(* Logix 5000 AddOnInstructionDefinition export YAI_Assy_151_116_EIP_Hz; software revision 21.03 *)

ADD_ON_INSTRUCTION YAI_Assy_151_116_EIP_Hz   (* revision 1.1, vendor Yaskawa America, Inc. *)
// YAI Assembly 151 and 116
// Help:
// This add-on instruction is for use with input assemblie 166 and output assemblies 116.
// Node_Input_Assy is defined as the node's input assembly integer array.
// Node_Output_Assy is defined as the node's output assembly integer array.
// Torque limit/reference, torque compensation and torque output variables are only available with A1000.
VAR_IN_OUT
   Node_Input_Assy : AB:ETHERNET_MODULE_INT_8Bytes:I:0; {required}   // Input assembly words
   Node_Output_Assy : AB:ETHERNET_MODULE_INT_44Bytes:O:0; {required}   // Output assembly words
END_VAR
VAR_INPUT
   RunFwd : BOOL; {visible}   // Forward run command
   RunRev : BOOL; {visible}   // Reverse run command
   MFI_3 : BOOL; {visible}   // Multi-function input 3
   MFI_4 : BOOL; {visible}   // Multi-function input 4
   MFI_5 : BOOL; {visible}   // Multi-function input 5
   MFI_6 : BOOL; {visible}   // Multi-function input 6
   MFI_7 : BOOL; {visible}   // Multi-function input 7
   MFI_8 : BOOL; {visible}   // Multi-function input 8
   External_Fault : BOOL;   // External fault command (EF0)
   FaultReset : BOOL; {visible}   // Fault reset command
   MFO_1 : BOOL; {visible}   // Multi-function output (M1-M2 for A/P1000, MA/MB/MC for V1000)
   MFO_2 : BOOL; {visible}   // Multi-function output (M3-M4 for A/P1000, P1 for V1000)
   MFO_3 : BOOL; {visible}   // Multi-function output (M5-M6 for A/P1000, P2 for V1000)
   Freq_Ref : REAL; {visible}   // Frequency reference command in Hz (xx.xx resolution)
   Torq_Ref_Limit : REAL; {visible}   // Torque reference/limit (A1000 only)
   Torq_Comp : REAL; {visible}   // Torque compensation command (A1000 only)
   Analog_Output_1 : REAL;   // Analog output 1 level command
   Analog_Output_2 : REAL;   // Analog output 2 level command
   Digital_Output_1 : BOOL;   // Digital output 1 activation - M1-M2
   Digital_Output_2 : BOOL;   // Digital output 2 activation - M3-M4
   Digital_Output_3 : BOOL;   // Digital output 3 activation - M5-M6
   Digital_Output_Fault_Enable : BOOL;   // Bit to enable control of fault output relay over the network
   Digital_Output_Fault : BOOL;   // Fault relay activation - MA-MB-MC
   Custom_Out_1 : INT; {visible}   // Custom output 1 - F7-23
   Custom_Out_2 : INT; {visible}   // Custom output 2 - F7-24
   Custom_Out_3 : INT; {visible}   // Custom output 3 - F7-25
   Custom_Out_4 : INT;   // Custom output 4 - F7-26
   Custom_Out_5 : INT;   // Custom output 5 - F7-27
   Custom_Out_6 : INT;   // Custom output 6 - F7-28
   Custom_Out_7 : INT;   // Custom output 7 - F7-29
   Custom_Out_8 : INT;   // Custom output 8 - F7-30
   Custom_Out_9 : INT;   // Custom output 9 - F7-31
   Custom_Out_10 : INT;   // Custom output 10 - F7-32
END_VAR
VAR_OUTPUT
   RunningRev : BOOL; {access Read Only, visible}   // Drive running reverse status bit
   At_Speed : BOOL; {access Read Only, visible}   // Drive at commanded speed status bit
   Ready : BOOL; {access Read Only, visible}   // Drive ready status bit
   Alarm : BOOL; {access Read Only, visible}   // Drive alarm status bit
   Faulted : BOOL; {access Read Only, visible}   // Drive faulted status bit
   Output_Freq : REAL; {access Read Only, visible}   // Drive output frequency in Hz (xx.xx resolution)
   Warning : BOOL; {access Read Only}
   RunningFwd : BOOL; {access Read Only}
END_VAR
VAR_INPUT
   Motor_Rated_Torq : REAL;
END_VAR
VAR_OUTPUT
   Running : BOOL; {access Read Only}
   ZSP : BOOL; {access Read Only}
   Reset : BOOL; {access Read Only}
   OPE : BOOL; {access Read Only}
   UV : BOOL; {access Read Only}
   MFO_1_Status : BOOL; {access Read Only}
   MFO_2_Status : BOOL; {access Read Only}
   MFO_3_Status : BOOL; {access Read Only}
   ZSV : BOOL; {access Read Only}
   Torque_Actual : REAL; {access Read Only}
   Output_Current : REAL; {access Read Only}
END_VAR
VAR_INPUT
   Net_Ref : BOOL;
   Net_Control : BOOL;
END_VAR
VAR_OUTPUT
   NetCtrlStatus : BOOL; {access Read Only}
END_VAR
VAR
   FRef_Convert : DINT;
   FOut_Convert : REAL;
   FOut_Temp : REAL;
   TRef_Convert : INT;
   TComp_Convert : INT;
   IOut_Temp : REAL;
   IOut_Convert : REAL;
   AO1_Convert : INT;
   AO2_Convert : INT;
   Motor_Speed_Temp : REAL;
   Motor_Speed_Convert : REAL;
   Freq_Cmd_Temp : REAL;
   Freq_Cmd_Convert : REAL;
   AI1_Temp : REAL;
   AI1_Convert : REAL;
   DriveStatusTempBits : INT;
   TOut_Temp : REAL;
   TOut_Convert : REAL;
END_VAR

ROUTINE Logic   (* ladder *)
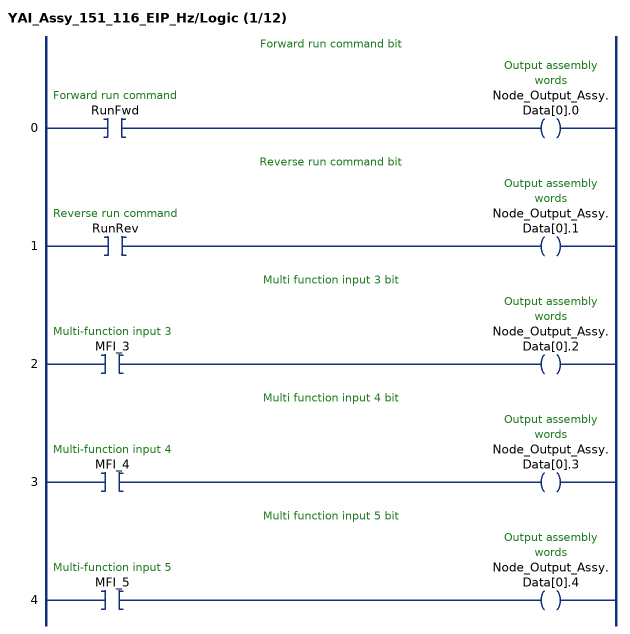
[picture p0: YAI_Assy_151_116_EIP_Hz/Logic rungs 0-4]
   // Forward run command bit
   0: XIC(RunFwd)OTE(Node_Output_Assy.Data[0].0);
   // Reverse run command bit
   1: XIC(RunRev)OTE(Node_Output_Assy.Data[0].1);
   // Multi function input 3 bit
   2: XIC(MFI_3)OTE(Node_Output_Assy.Data[0].2);
   // Multi function input 4 bit
   3: XIC(MFI_4)OTE(Node_Output_Assy.Data[0].3);
   // Multi function input 5 bit
   4: XIC(MFI_5)OTE(Node_Output_Assy.Data[0].4);
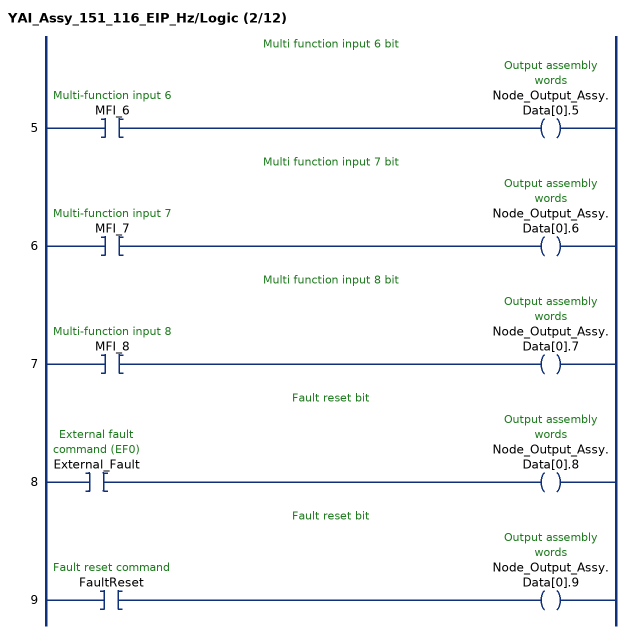
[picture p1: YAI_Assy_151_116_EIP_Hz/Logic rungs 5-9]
   // Multi function input 6 bit
   5: XIC(MFI_6)OTE(Node_Output_Assy.Data[0].5);
   // Multi function input 7 bit
   6: XIC(MFI_7)OTE(Node_Output_Assy.Data[0].6);
   // Multi function input 8 bit
   7: XIC(MFI_8)OTE(Node_Output_Assy.Data[0].7);
   // Fault reset bit
   8: XIC(External_Fault)OTE(Node_Output_Assy.Data[0].8);
   // Fault reset bit
   9: XIC(FaultReset)OTE(Node_Output_Assy.Data[0].9);
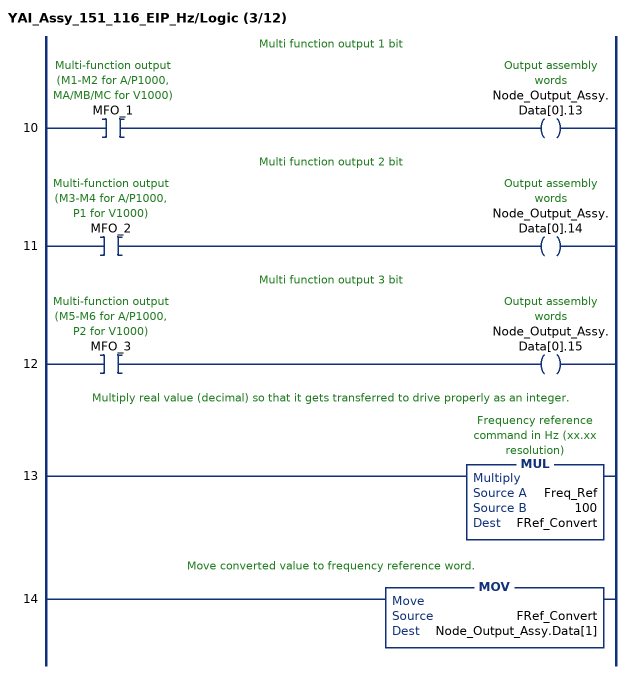
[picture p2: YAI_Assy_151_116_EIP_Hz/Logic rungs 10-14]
   // Multi function output 1 bit
   10: XIC(MFO_1)OTE(Node_Output_Assy.Data[0].13);
   // Multi function output 2 bit
   11: XIC(MFO_2)OTE(Node_Output_Assy.Data[0].14);
   // Multi function output 3 bit
   12: XIC(MFO_3)OTE(Node_Output_Assy.Data[0].15);
   // Multiply real value (decimal) so that it gets transferred to drive properly as an integer.
   13: MUL(Freq_Ref,100,FRef_Convert);
   // Move converted value to frequency reference word.
   14: MOV(FRef_Convert,Node_Output_Assy.Data[1]);
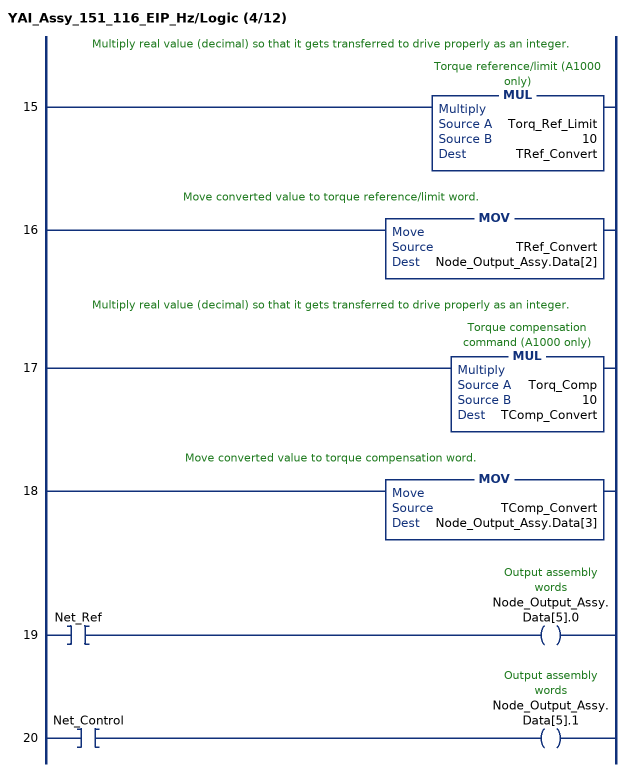
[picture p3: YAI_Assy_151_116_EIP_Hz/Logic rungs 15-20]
   // Multiply real value (decimal) so that it gets transferred to drive properly as an integer.
   15: MUL(Torq_Ref_Limit,10,TRef_Convert);
   // Move converted value to torque reference/limit word.
   16: MOV(TRef_Convert,Node_Output_Assy.Data[2]);
   // Multiply real value (decimal) so that it gets transferred to drive properly as an integer.
   17: MUL(Torq_Comp,10,TComp_Convert);
   // Move converted value to torque compensation word.
   18: MOV(TComp_Convert,Node_Output_Assy.Data[3]);
   19: XIC(Net_Ref)OTE(Node_Output_Assy.Data[5].0);
   20: XIC(Net_Control)OTE(Node_Output_Assy.Data[5].1);
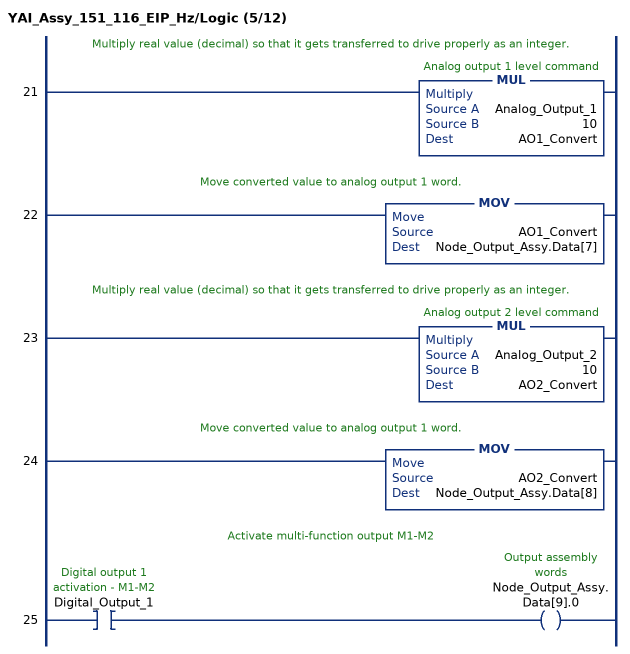
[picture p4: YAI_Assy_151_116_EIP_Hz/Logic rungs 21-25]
   // Multiply real value (decimal) so that it gets transferred to drive properly as an integer.
   21: MUL(Analog_Output_1,10,AO1_Convert);
   // Move converted value to analog output 1 word.
   22: MOV(AO1_Convert,Node_Output_Assy.Data[7]);
   // Multiply real value (decimal) so that it gets transferred to drive properly as an integer.
   23: MUL(Analog_Output_2,10,AO2_Convert);
   // Move converted value to analog output 1 word.
   24: MOV(AO2_Convert,Node_Output_Assy.Data[8]);
   // Activate multi-function output M1-M2
   25: XIC(Digital_Output_1)OTE(Node_Output_Assy.Data[9].0);
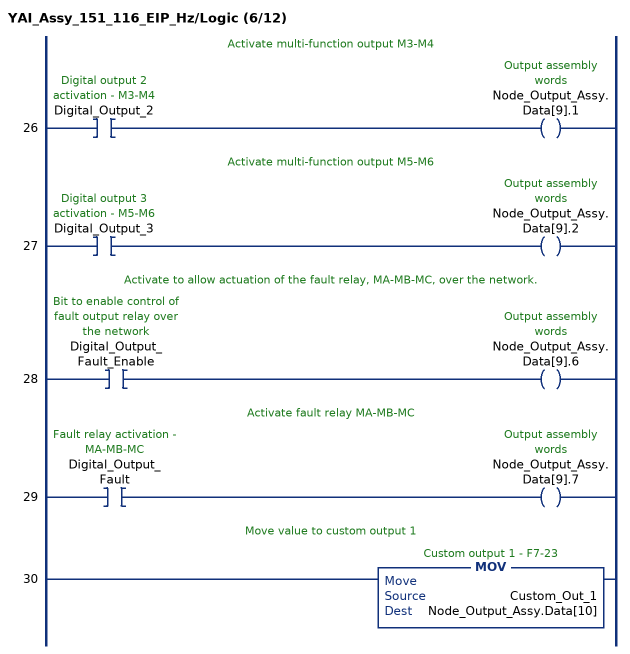
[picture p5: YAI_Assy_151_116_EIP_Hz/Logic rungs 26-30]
   // Activate multi-function output M3-M4
   26: XIC(Digital_Output_2)OTE(Node_Output_Assy.Data[9].1);
   // Activate multi-function output M5-M6
   27: XIC(Digital_Output_3)OTE(Node_Output_Assy.Data[9].2);
   // Activate to allow actuation of the fault relay, MA-MB-MC, over the network.
   28: XIC(Digital_Output_Fault_Enable)OTE(Node_Output_Assy.Data[9].6);
   // Activate fault relay MA-MB-MC
   29: XIC(Digital_Output_Fault)OTE(Node_Output_Assy.Data[9].7);
   // Move value to custom output 1
   30: MOV(Custom_Out_1,Node_Output_Assy.Data[10]);
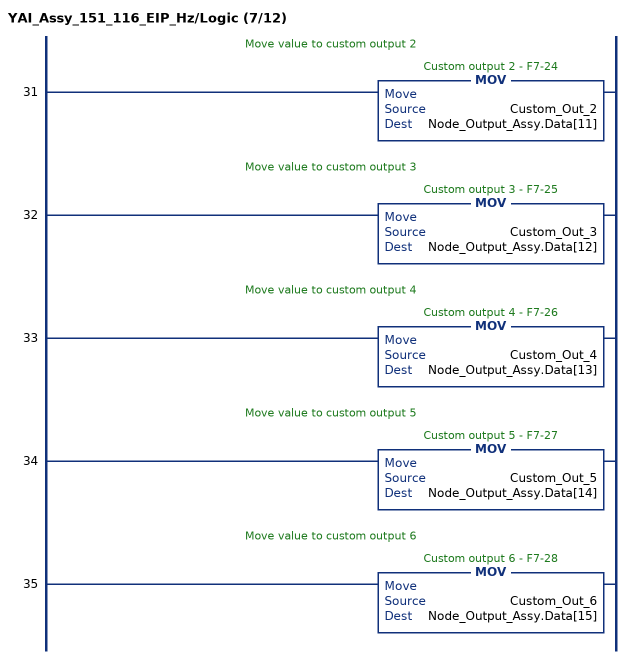
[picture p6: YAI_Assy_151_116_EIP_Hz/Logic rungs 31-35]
   // Move value to custom output 2
   31: MOV(Custom_Out_2,Node_Output_Assy.Data[11]);
   // Move value to custom output 3
   32: MOV(Custom_Out_3,Node_Output_Assy.Data[12]);
   // Move value to custom output 4
   33: MOV(Custom_Out_4,Node_Output_Assy.Data[13]);
   // Move value to custom output 5
   34: MOV(Custom_Out_5,Node_Output_Assy.Data[14]);
   // Move value to custom output 6
   35: MOV(Custom_Out_6,Node_Output_Assy.Data[15]);
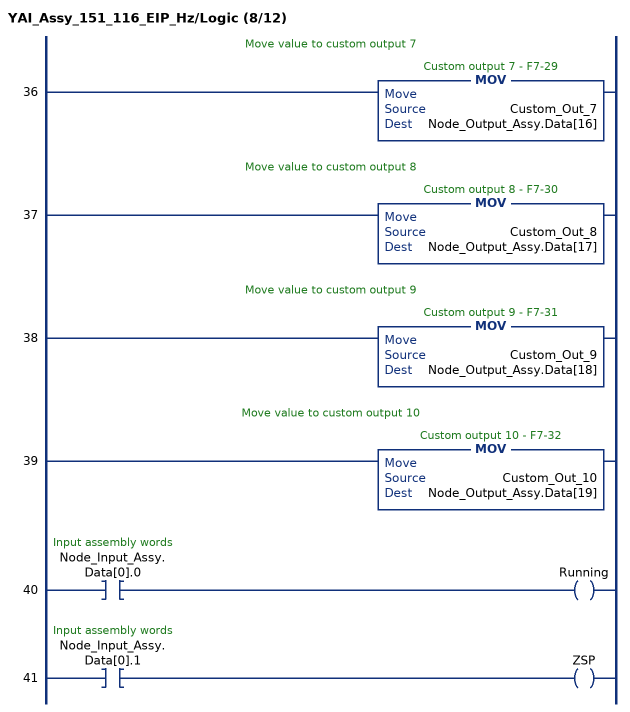
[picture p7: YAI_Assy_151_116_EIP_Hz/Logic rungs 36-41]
   // Move value to custom output 7
   36: MOV(Custom_Out_7,Node_Output_Assy.Data[16]);
   // Move value to custom output 8
   37: MOV(Custom_Out_8,Node_Output_Assy.Data[17]);
   // Move value to custom output 9
   38: MOV(Custom_Out_9,Node_Output_Assy.Data[18]);
   // Move value to custom output 10
   39: MOV(Custom_Out_10,Node_Output_Assy.Data[19]);
   40: XIC(Node_Input_Assy.Data[0].0)OTE(Running);
   41: XIC(Node_Input_Assy.Data[0].1)OTE(ZSP);
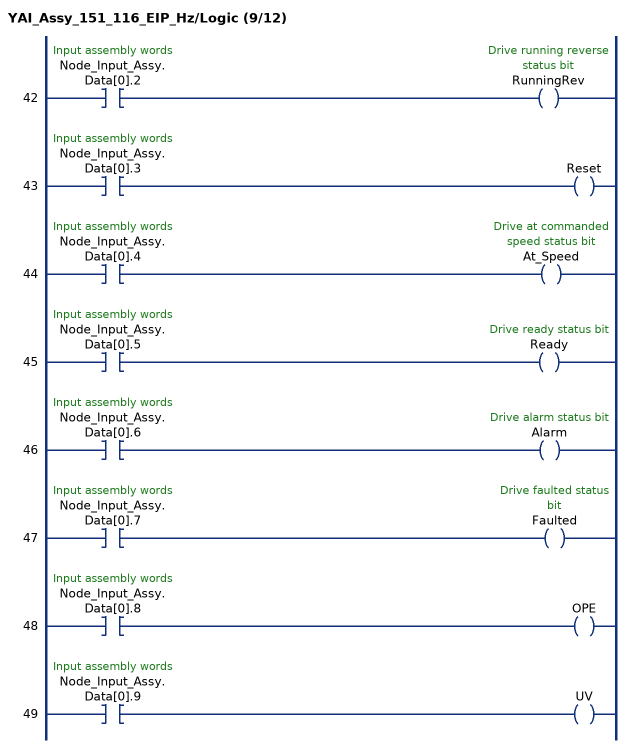
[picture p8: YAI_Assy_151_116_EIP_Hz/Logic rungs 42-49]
   42: XIC(Node_Input_Assy.Data[0].2)OTE(RunningRev);
   43: XIC(Node_Input_Assy.Data[0].3)OTE(Reset);
   44: XIC(Node_Input_Assy.Data[0].4)OTE(At_Speed);
   45: XIC(Node_Input_Assy.Data[0].5)OTE(Ready);
   46: XIC(Node_Input_Assy.Data[0].6)OTE(Alarm);
   47: XIC(Node_Input_Assy.Data[0].7)OTE(Faulted);
   48: XIC(Node_Input_Assy.Data[0].8)OTE(OPE);
   49: XIC(Node_Input_Assy.Data[0].9)OTE(UV);
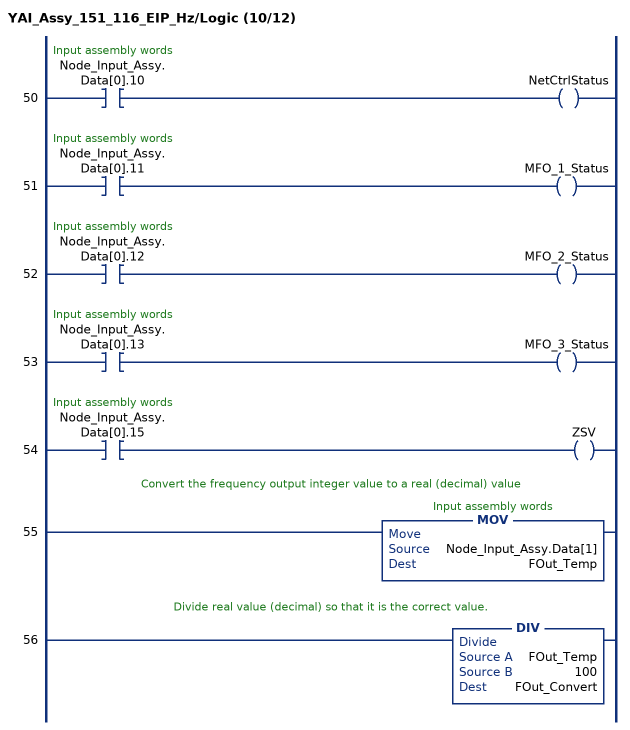
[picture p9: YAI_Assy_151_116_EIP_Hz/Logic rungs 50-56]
   50: XIC(Node_Input_Assy.Data[0].10)OTE(NetCtrlStatus);
   51: XIC(Node_Input_Assy.Data[0].11)OTE(MFO_1_Status);
   52: XIC(Node_Input_Assy.Data[0].12)OTE(MFO_2_Status);
   53: XIC(Node_Input_Assy.Data[0].13)OTE(MFO_3_Status);
   54: XIC(Node_Input_Assy.Data[0].15)OTE(ZSV);
   // Convert the frequency output integer value to a real (decimal) value
   55: MOV(Node_Input_Assy.Data[1],FOut_Temp);
   // Divide real value (decimal) so that it is the correct value.
   56: DIV(FOut_Temp,100,FOut_Convert);
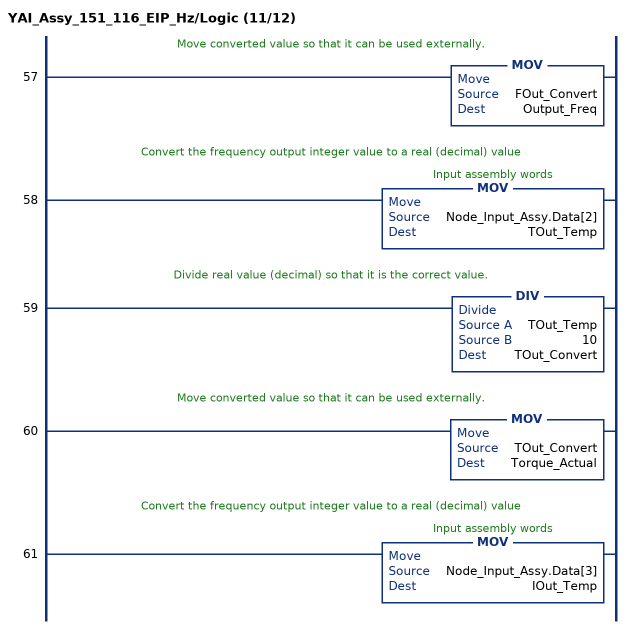
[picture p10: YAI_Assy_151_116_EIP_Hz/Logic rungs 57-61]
   // Move converted value so that it can be used externally.
   57: MOV(FOut_Convert,Output_Freq);
   // Convert the frequency output integer value to a real (decimal) value
   58: MOV(Node_Input_Assy.Data[2],TOut_Temp);
   // Divide real value (decimal) so that it is the correct value.
   59: DIV(TOut_Temp,10,TOut_Convert);
   // Move converted value so that it can be used externally.
   60: MOV(TOut_Convert,Torque_Actual);
   // Convert the frequency output integer value to a real (decimal) value
   61: MOV(Node_Input_Assy.Data[3],IOut_Temp);
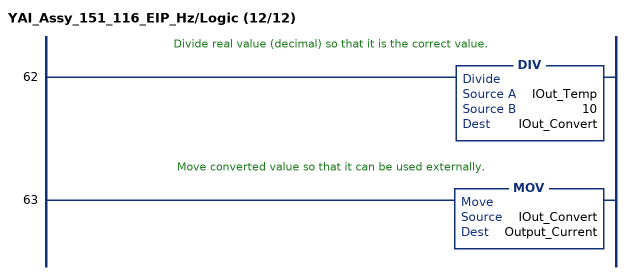
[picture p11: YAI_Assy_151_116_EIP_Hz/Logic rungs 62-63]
   // Divide real value (decimal) so that it is the correct value.
   62: DIV(IOut_Temp,10,IOut_Convert);
   // Move converted value so that it can be used externally.
   63: MOV(IOut_Convert,Output_Current);
END_ROUTINE
END_ADD_ON_INSTRUCTION
